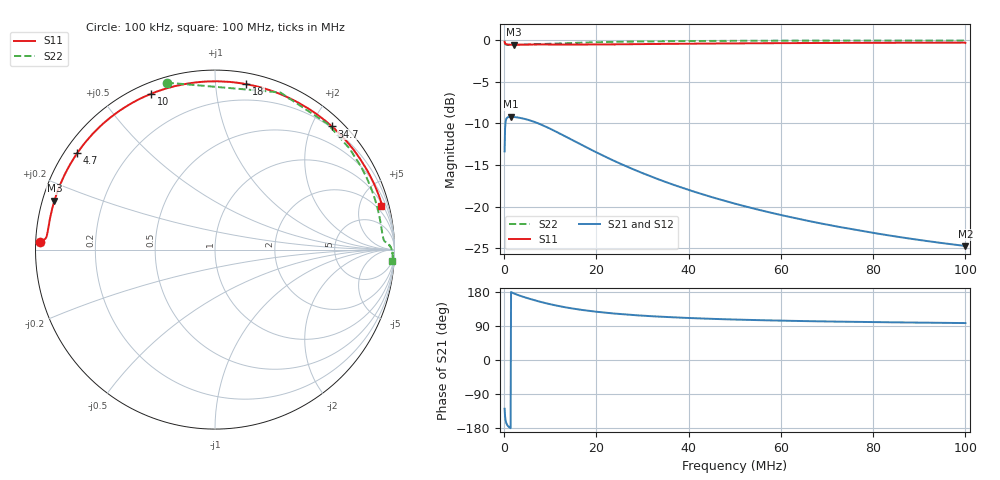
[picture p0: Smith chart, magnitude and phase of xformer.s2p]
# Hz S RI R 50.0
! written by SimSmith version 18.3h
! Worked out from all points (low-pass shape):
!   1000 points, 100 kHz to 100 MHz, reference 50 ohm
!   highest |S21| = -9.22 dB at 1.5 MHz (marker M1); lowest = -24.7 dB at 100 MHz (marker M2)
!   |S21| within 3 dB of the highest: 142.4 kHz to 15.5 MHz (15.36 MHz wide, 196 % of centre)
!   lowest |S11| = -0.6 dB at 2.2 MHz (marker M3), VSWR 29.87, Z = 1.71 + j7.45 ohm
!   |S11| at or under -10 dB: nowhere
!   |S22| runs from -0.6 to -0.1 dB; largest |S21 - S12| = 0.0057
!   S11 on the Smith chart (normalised r, x): 100 kHz: 0.01, +0.02; 4.7 MHz: 0.04, +0.31; 10 MHz: 0.05, +0.67; 18 MHz: 0.08, +1.21; 34.7 MHz: 0.18, +2.32; 100 MHz: 1.22, +7.50
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100000  -0.9751 0.044  -0.1342 -0.1675  -0.1351 -0.17  -0.2692 0.9304
700000  -0.9323 0.0995  -0.3395 -0.0465  -0.3451 -0.0472  0.8677 0.3472
800000  -0.9304 0.1105  -0.342 -0.0368  -0.3476 -0.0373  0.8825 0.3069
1000000  -0.9268 0.1333  -0.3446 -0.0218  -0.3503 -0.0217  0.9005 0.2491
1500000  -0.9155 0.1916  -0.3461 0.00393  -0.3517 0.00478  0.9188 0.1704
2200000  -0.8945 0.2729  -0.3438 0.0287  -0.3491 0.0304  0.9273 0.1202
4700000  -0.7675 0.5374  -0.3226 0.0892  -0.3262 0.0925  0.937 0.065
7300000  -0.5747 0.7421  -0.2877 0.1324  -0.2897 0.1362  0.9419 0.0497
1e7  -0.354 0.8691  -0.2464 0.1592  -0.2468 0.1627  0.9473 0.0439
1.31e7  -0.1188 0.93  -0.2017 0.1724  -0.2012 0.1752  0.9544 0.0397
1.68e7  0.1121 0.9311  -0.1579 0.1737  -0.1569 0.1756  0.9622 0.0342
1.8e7  0.1753 0.9218  -0.146 0.1722  -0.1449 0.1739  0.9645 0.0322
2.13e7  0.3214 0.8825  -0.1185 0.1653  -0.1174 0.1665  0.9696 0.0268
2.48e7  0.4406 0.8311  -0.0961 0.156  -0.0951 0.1568  0.9738 0.0218
2.89e7  0.5459 0.7691  -0.0765 0.1447  -0.0755 0.1452  0.9779 0.0157
3.34e7  0.6311 0.7039  -0.0608 0.1329  -0.06 0.1332  0.9811 0.00942
3.47e7  0.6513 0.6862  -0.0571 0.1298  -0.0564 0.13  0.9818 0.00763
4.17e7  0.7358 0.6001  -0.0417 0.1145  -0.0412 0.1146  0.985 -0.0014
5.01e7  0.8012 0.5158  -0.03 0.0998  -0.0296 0.0999  0.9873 -0.0111
6.67e7  0.8729 0.394  -0.0175 0.0795  -0.0172 0.0796  0.9899 -0.0292
8.34e7  0.9097 0.3096  -0.0111 0.0664  -0.0109 0.0665  0.9901 -0.0457
1e8  0.9274 0.2451  -0.00751 0.0576  -0.00733 0.0576  0.985 -0.0654
